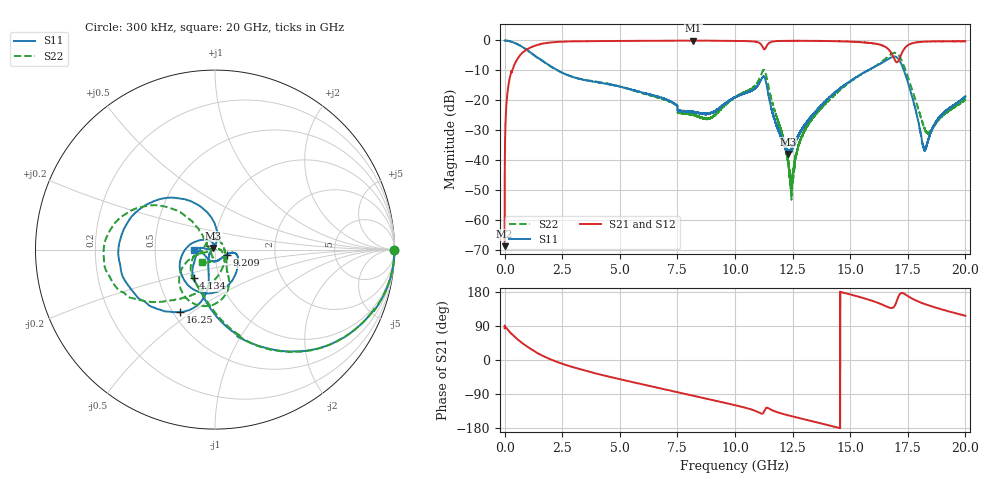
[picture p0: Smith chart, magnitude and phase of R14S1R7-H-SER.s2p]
!{R14S1R7}
!Johanson Technology Inc.
!www.johansontechnology.com
!Test Board Conditions:
!Substrate Type  RO4350B
!Substrate Thickness  20 mil
!Substrate Dk  3.66
!TL Type: GCPW
!TL Trace Width  36 mil
!TL Gap  12 mil
!Electrode orientation  Horizontal
!DUT TOPOLOGY	SERIES
!Mounting Pad LxW  26x36 mil
! Created Wed Nov 25 17:33:21 2020
! 2 Port Network Data from SP1.SP block
! freq  magS11  angS11  magS21  angS21  magS12  angS12  magS22  angS22
# khz S ma R 50
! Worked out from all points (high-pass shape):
!   20001 points, 300 kHz to 20 GHz, reference 50 ohm
!   highest |S21| = -0.06 dB at 8.189 GHz (marker M1); lowest = -68.6 dB at 300 kHz (marker M2)
!   |S21| within 3 dB of the highest: 950.6 MHz to 16.68 GHz (15.73 GHz wide, 178 % of centre); 17.32 GHz to end of sweep
!   lowest |S11| = -37.8 dB at 12.31 GHz (marker M3), VSWR 1.03, Z = 49.1 + j0.854 ohm
!   |S11| at or under -10 dB: 2.309 GHz to 15.76 GHz (13.45 GHz wide, 149 % of centre); 15.76043 GHz to 15.7624 GHz (1.979 MHz wide, 0.0126 % of centre); 17.33 GHz to end of sweep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
!   |S22| runs from -53.1 to 0.0 dB; largest |S21 - S12| = 0.016
!   S11 on the Smith chart (normalised r, x): 300 kHz: open; 4.134 GHz: 0.75, -0.25; 9.209 GHz: 1.13, -0.07; 16.25 GHz: 0.54, -0.45; 20 GHz: 0.79, -0.00
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300  0.9961 -0.2  0.0003729 83.8  0.0003192 83.4  0.9985 -0.0
132300  0.9893 -9.6  0.1433 80.2  0.1441 80.3  0.9887 -9.6
495300  0.8887 -31.2  0.4478 58.2  0.4485 58.2  0.8882 -31.1
1673300  0.4495 -79.8  0.8894 10.6  0.8899 10.5  0.4485 -78.9
3334300  0.2248 -115.5  0.9705 -25.4  0.9695 -25.4  0.2272 -115.0
4134300  0.1979 -127.0  0.9758 -38.2  0.9758 -38.1  0.2011 -128.7
6667300  0.1159 -159.0  0.9878 -73.6  0.9879 -73.6  0.1117 -166.5
8189300  0.06477 -81.3  0.9932 -94.4  0.9912 -94.3  0.05783 75.9
9209300  0.07042 -24.5  0.9906 -108.2  0.9904 -108.3  0.06138 -19.8
1.00003e7  0.1135 -10.0  0.9844 -119.2  0.9839 -119.3  0.1129 -55.1
1.09823e7  0.1767 -49.0  0.9382 -136.8  0.9365 -136.7  0.2014 -67.2
1.12803e7  0.2448 -132.5  0.7112 -133.6  0.7109 -133.4  0.3202 -116.6
1.23063e7  0.01285 137.4  0.985 -145.9  0.9873 -145.8  0.009453 175.8
1.24753e7  0.01574 173.7  0.9846 -148.5  0.9879 -148.4  0.004422 69.7
1.28053e7  0.02865 -151.8  0.9868 -153.4  0.9865 -153.4  0.02071 10.0
1.33343e7  0.05588 -128.7  0.9834 -161.4  0.9854 -161.3  0.04764 -23.5
1.62523e7  0.3981 -119.3  0.8582 149.6  0.854 149.7  0.4108 -135.1
1.66673e7  0.4904 -144.4  0.7092 138.8  0.6962 138.8  0.5514 -151.7
1.72323e7  0.394 132.8  0.6056 176.8  0.5995 177.1  0.4675 149.2
1.82283e7  0.01506 128.7  0.9547 147.9  0.955 147.5  0.03407 173.0
1.88573e7  0.05199 175.6  0.9672 135.6  0.9643 135.8  0.04852 -105.0
2e7  0.1165 -179.9  0.9688 116.7  0.9658 116.9  0.1031 -136.4
